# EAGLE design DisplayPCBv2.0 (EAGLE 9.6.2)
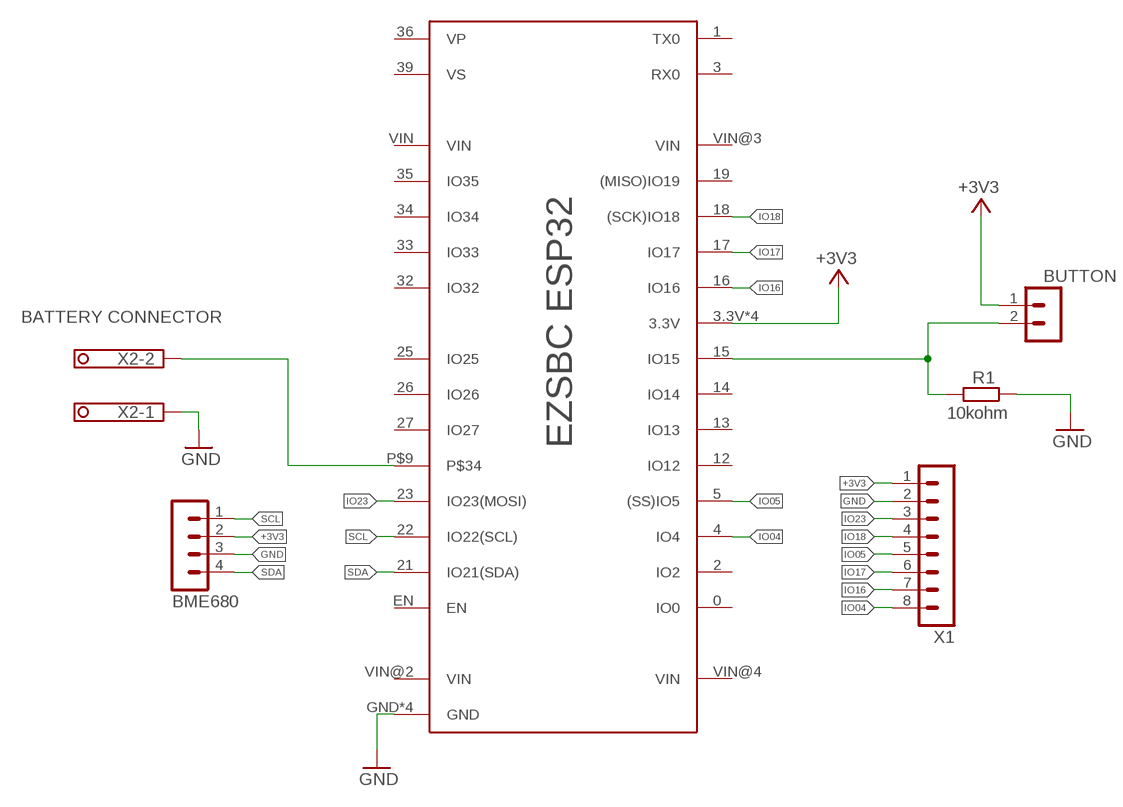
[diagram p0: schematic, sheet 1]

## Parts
BME680  B4B-PH-K-S  [B4B-PH-K-S]
BUTTON  B2B-PH-K-S  [B2B-PH-K-S]
R1  10kohm  R-EU_R0805  [R0805]
U$1  EZSBCESP32  [EZSBCBATPRO]
X1  B8B-PH-K-S  [B8B-PH-K-S]
X2  1751248  [1751248]

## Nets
+3V3: BME680.2 BUTTON.1 U$1.3.3V U$1.3.3V@2(3.3V) U$1.3.3V@4(3.3V) U$1.3.3V@5(3.3V) X1.1
GND: BME680.3 R1.1 U$1.GND U$1.GND@2(GND) U$1.GND@3(GND) U$1.GND@4(GND) X1.2 X2.1
IO04: U$1.4(IO4) X1.8
IO05: U$1.5((SS)IO5) X1.5
IO16: U$1.16(IO16) X1.7
IO17: U$1.17(IO17) X1.6
IO18: U$1.18((SCK)IO18) X1.4
IO23: U$1.23(IO23(MOSI)) X1.3
N$9: BUTTON.2 R1.2 U$1.15(IO15)
SCL: BME680.1 U$1.22(IO22(SCL))
SDA: BME680.4 U$1.21(IO21(SDA))
VBAT: U$1.P$9 X2.2
Unconnected: U$1.0(IO0) U$1.1(TX0) U$1.2(IO2) U$1.3(RX0) U$1.12(IO12) U$1.13(IO13) U$1.14(IO14) U$1.19((MISO)IO19) U$1.25(IO25) U$1.26(IO26) U$1.27(IO27) U$1.32(IO32) U$1.33(IO33) U$1.34(IO34) U$1.35(IO35) U$1.36(VP) U$1.39(VS) U$1.EN U$1.VIN U$1.VIN@2(VIN) U$1.VIN@3(VIN) U$1.VIN@4(VIN)

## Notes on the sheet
- BATTERY CONNECTOR

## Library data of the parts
BME680 = con-JSTPH:B4B-PH: JST PH series header 2.00mm pitch disconnectable crimp style connectors, vertical (side entry type), 4 pins
BUTTON = con-JSTPH:B2B-PH: JST PH series header 2.00mm pitch disconnectable crimp style connectors, vertical (side entry type), 2 pins
R1 = rcl:R-EU_: RESISTOR, European symbol; SPICEPREFIX: R
U$1 = EzbscBatESP32:EZSBCESP32
X1 = con-JSTPH:B8B-PH: JST PH series header 2.00mm pitch disconnectable crimp style connectors, vertical (side entry type), 8 pins
X2 = con-phoenix-350:1751248: MKDS 1/ 2-3,5 Printklemme; OC_FARNELL: unknown; OC_NEWARK: unknown

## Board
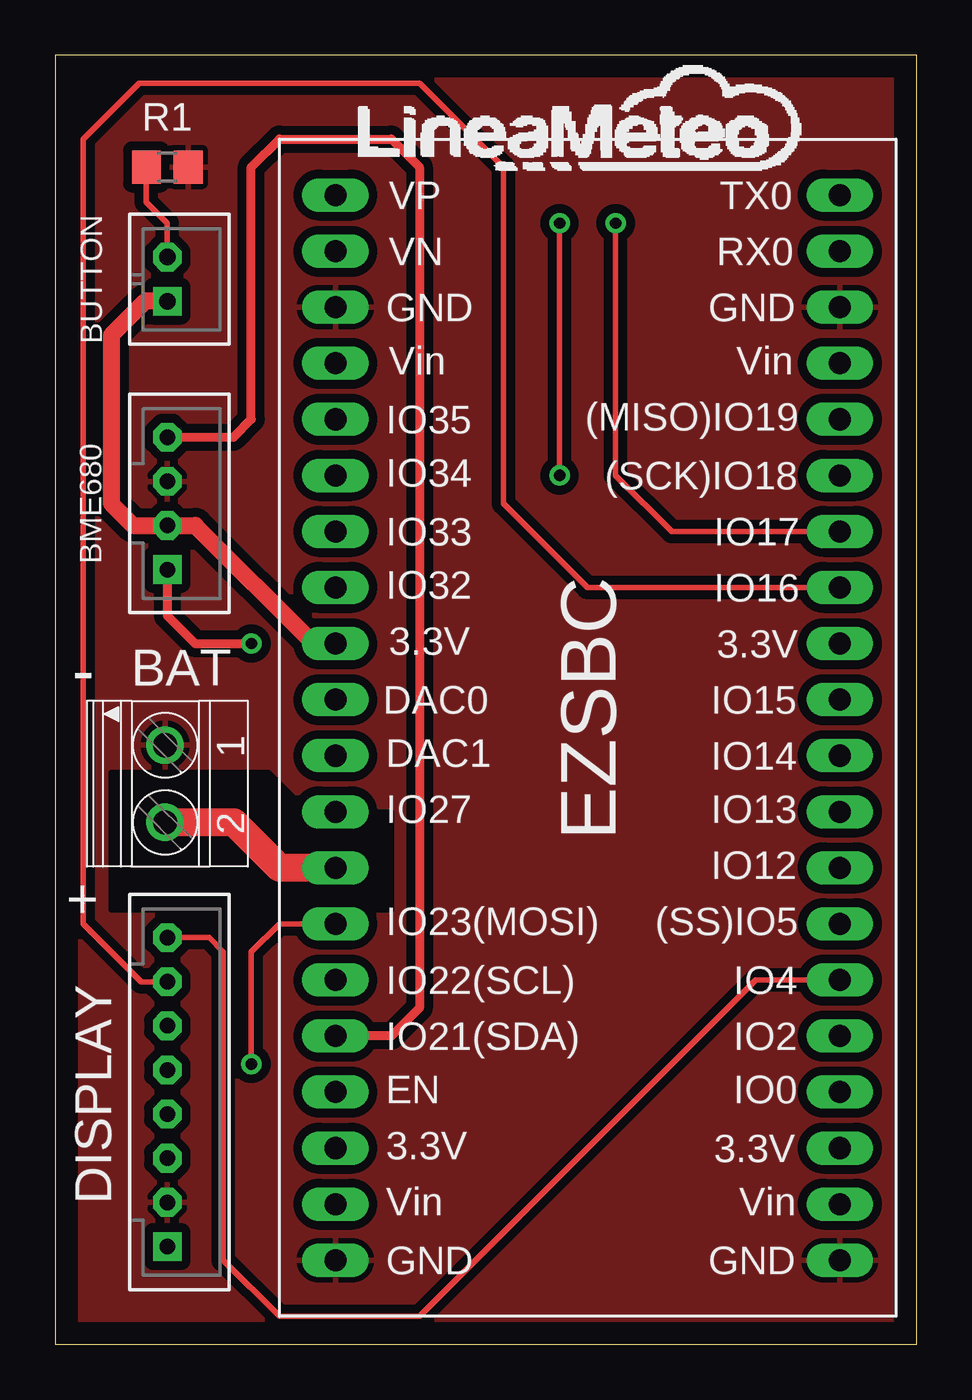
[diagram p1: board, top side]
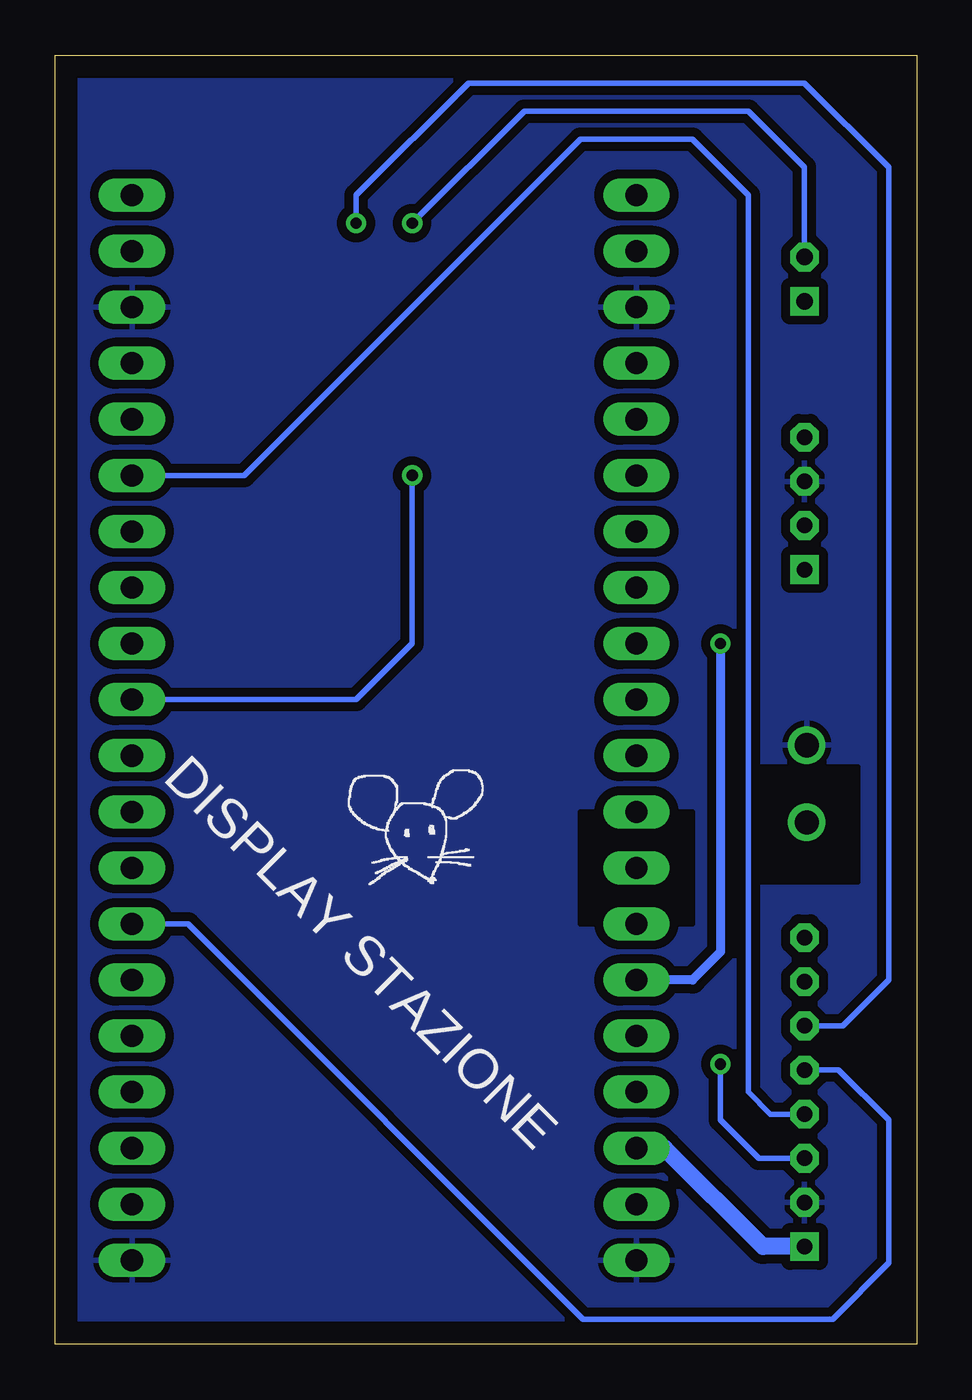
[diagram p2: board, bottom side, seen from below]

Size 39.04 x 58.41 mm. Coordinates in mm from the lower left corner, seen from the top.
Outline: 0,0 39.04,0 39.04,58.41 0,58.41 0,0
Copper layers (1*16): Top 0.035mm / dielectric 1.5mm / Bottom 0.035mm
Design rules "default": minimum track width 6mil, minimum drill 0.35mm, track to track 6mil, track to pad 6mil, pad to pad 6mil, via to via 6mil, smd to smd 6mil, copper to edge 40mil, drill to drill 6mil, minimum pad ring 10mil, minimum via ring 8mil, stop-mask expansion 4mil, vias tented up to drill 0mil, thermal gap 10mil

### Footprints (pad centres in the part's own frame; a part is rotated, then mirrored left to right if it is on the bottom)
B4B-PH-K-S = drill 0.7 pad 1.3 square: 1 3,0 | drill 0.7 pad 1.3 octagon: 2 1,0; 3 -1,0; 4 -3,0
B2B-PH-K-S = drill 0.75 pad 1.3 square: 1 1,0 | drill 0.75 pad 1.3 octagon: 2 -1,0
R0805 = smd 1.3 x 1.5: 1 -0.95,0; 2 0.95,0
EZSBCBATPRO = drill 1 long: 0 7.62,2.54; 1 7.62,43.18; 2 7.62,5.08; 3 7.62,40.64; 3.3V -15.24,22.86; 3.3V@2 -15.24,0; 3.3V@4 7.62,22.86; 3.3V@5 7.62,0; 4 7.62,7.62; 5 7.62,10.16; 12 7.62,12.7; 13 7.62,15.24; 14 7.62,17.78; 15 7.62,20.32; 16 7.62,25.4; 17 7.62,27.94; 18 7.62,30.48; 19 7.62,33.02; 21 -15.24,5.08; 22 -15.24,7.62; 23 -15.24,10.16; 25 -15.24,20.32; 26 -15.24,17.78; 27 -15.24,15.24; 32 -15.24,25.4; 33 -15.24,27.94; 34 -15.24,30.48; 35 -15.24,33.02; 36 -15.24,43.18; 39 -15.24,40.64; EN -15.24,2.54; GND -15.24,38.1; GND@2 -15.24,-5.08; GND@3 7.62,38.1; GND@4 7.62,-5.08; P$9 -15.24,12.7; VIN -15.24,35.56; VIN@2 -15.24,-2.54; VIN@3 7.62,35.56; VIN@4 7.62,-2.54
B8B-PH-K-S = drill 0.7 pad 1.3 square: 1 7,0 | drill 0.7 pad 1.3 octagon: 2 5,0; 3 3,0; 4 1,0; 5 -1,0; 6 -3,0; 7 -5,0; 8 -7,0
1751248 = drill 1.1 pad 1.7: 1 -1.75,-0.1; 2 1.75,-0.1

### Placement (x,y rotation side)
BME680  5.08,38.1 270 top
BUTTON  5.08,48.26 270 top
R1  5.08,53.34 180 top
U$1  27.94,8.89 0 top
X1  5.08,11.43 270 top
X2  5.08,25.4 270 top

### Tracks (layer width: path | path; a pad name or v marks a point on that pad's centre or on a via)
+3V3
  Top 0.762: BUTTON.1 4.08,47.26 2.54,45.72 2.54,38.1 3.54,37.1 BME680.2 6.35,37.1 11.7,31.75 U$1.3.3V
  Bottom 0.762: X1.1 6.97,4.43 11.43,8.89 U$1.3.3V@2
GND
  pour Top (isolate 0.406, rank 2): 0,58.42 39.37,58.42 39.37,0 0,0
  pour Bottom (isolate 0.406, rank 2): 0,58.42 39.37,58.42 39.37,0 0,0
IO04
  Top 0.254: X1.8 6.97,18.43 7.62,17.78 7.62,3.81 10.16,1.27 16.51,1.27 31.75,16.51 U$1.4
IO05
  Bottom 0.254: X1.5 3.54,12.43 1.27,10.16 1.27,3.68 3.81,1.14 15.11,1.14 33.02,19.05 U$1.5
IO16
  Top 0.254: X1.7 3.89,16.43 1.27,19.05 1.27,54.61 3.81,57.15 16.51,57.15 20.32,53.34 20.32,38.1 24.13,34.29 U$1.16
IO17  (via drill 0.51)
  Top 0.254: v25.4,50.8 25.4,39.37 27.94,36.83 U$1.17
  Bottom 0.254: X1.6 3.35,14.43 1.27,16.51 1.27,53.34 5.08,57.15 20.32,57.15 25.4,52.07 v25.4,50.8
IO18
  Bottom 0.254: X1.4 6.62,10.43 7.62,11.43 7.62,52.07 10.16,54.61 15.24,54.61 30.48,39.37 U$1.18
IO23  (via drill 0.51)
  Top 0.254: U$1.23 10.16,19.05 8.89,17.78 v8.89,12.7
  Bottom 0.254: X1.3 7.16,8.43 8.89,10.16 v8.89,12.7
N$9  (via drill 0.51)
  Top 0.254: R1.2 4.13,51.75 5.08,50.8 BUTTON.2 | v22.86,50.8 v22.86,39.37
  Bottom 0.254: BUTTON.2 5.08,53.34 7.62,55.88 17.78,55.88 v22.86,50.8 | v22.86,39.37 22.86,31.75 25.4,29.21 U$1.15
NOGND
  cutout Top (isolate 0.406): 2.54,25.91 9.65,25.91 11.43,24.13 15.24,24.13 15.24,19.68 2.54,19.68
SCL  (via drill 0.51)
  Top 0.406: BME680.1 5.08,33.02 6.35,31.75 v8.89,31.75
  Bottom 0.406: U$1.22 10.16,16.51 8.89,17.78 v8.89,31.75
SDA
  Top 0.406: U$1.21 15.24,13.97 16.51,15.24 16.51,53.34 15.24,54.61 10.16,54.61 8.89,53.34 8.89,41.91 8.08,41.1 BME680.4
VBAT
  Top 1.27: U$1.P$9 10.16,21.59 8.1,23.65 X2.2
  cutout Bottom: 10.16,24.13 15.24,24.13 15.24,19.05 10.16,19.05
  cutout Bottom: 2.67,26.16 6.98,26.16 6.98,20.95 2.67,20.95

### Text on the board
tPlace: BAT | - | + | DISPLAY
bPlace: DISPLAY STAZIONE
